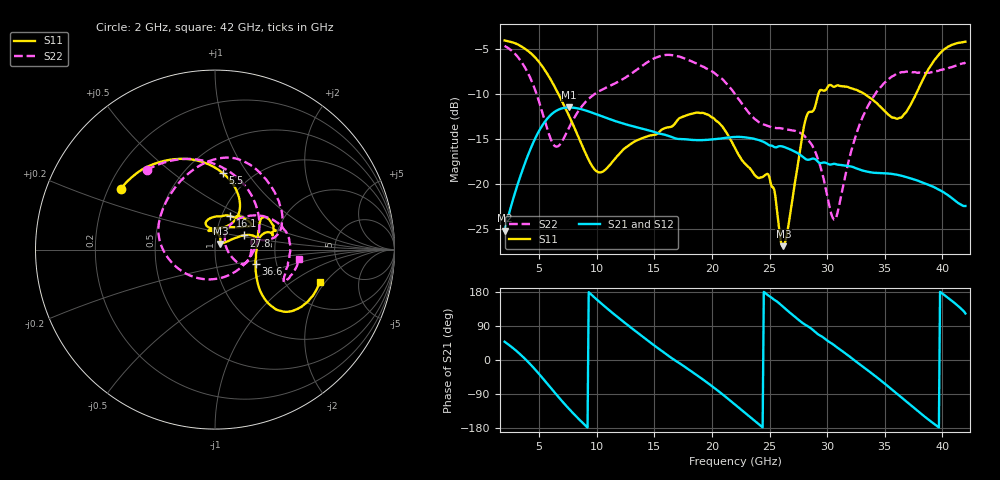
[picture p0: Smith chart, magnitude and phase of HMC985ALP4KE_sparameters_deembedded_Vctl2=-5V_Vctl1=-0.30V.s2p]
!s2p File: Measurements: S11, S21, S12, S22
# GHz S dB R 50.0
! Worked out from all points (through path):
!   401 points, 2 GHz to 42 GHz, reference 50 ohm
!   highest |S21| = -11.51 dB at 7.6 GHz (marker M1); lowest = -25.2 dB at 2 GHz (marker M2)
!   lowest |S11| = -26.9 dB at 26.2 GHz (marker M3), VSWR 1.09, Z = 52.9 + j3.6 ohm
!   |S11| at or under -10 dB: 6.664 GHz to 29.24 GHz (22.58 GHz wide, 126 % of centre); 33.21 GHz to 37.73 GHz (4.512 GHz wide, 12.7 % of centre)
!   |S22| runs from -24.0 to -4.7 dB; largest |S21 - S12| = 0.00026
!   S11 on the Smith chart (normalised r, x): 2 GHz: 0.25, +0.28; 5.5 GHz: 0.75, +0.78; 16.1 GHz: 1.10, +0.43; 27.8 GHz: 1.36, +0.22; 36.6 GHz: 1.56, -0.26; 42 GHz: 3.05, -1.80
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2  -4.08 147.2  -25.19 48.2  -25.19 48.2  -4.68 130.7
3.6  -4.86 120.5  -18.29 8.1  -18.29 8.1  -6.73 85.3
5.5  -7.38 84.0  -13.09 -55.1  -13.10 -55.1  -13.04 2.1
6.5  -9.59 67.0  -11.87 -91.4  -11.87 -91.4  -15.87 -71.2
7.6  -12.47 56.5  -11.51 -129.3  -11.51 -129.3  -13.74 -137.6
8.7  -15.66 58.8  -11.72 -163.6  -11.73 -163.6  -11.39 -171.4
10.2  -18.72 87.3  -12.37 154.2  -12.38 154.2  -9.71 164.3
11.9  -16.75 110.0  -13.15 111.1  -13.15 111.1  -8.64 141.1
15.4  -14.27 76.5  -14.41 29.3  -14.42 29.3  -5.86 87.2
16.1  -13.74 65.2  -14.61 13.8  -14.62 13.8  -5.68 78.5
19.4  -12.21 34.5  -15.12 -55.5  -15.13 -55.5  -7.10 35.6
22  -16.00 52.1  -14.79 -117.5  -14.79 -117.5  -10.03 10.5
24.9  -18.95 102.8  -15.65 170.1  -15.66 170.1  -13.60 13.0
26.2  -26.91 48.7  -15.87 139.6  -15.88 139.6  -13.88 -1.7
27.8  -15.01 26.4  -16.91 99.2  -16.91 99.2  -14.45 -22.7
28.7  -11.98 12.4  -17.20 81.0  -17.20 81.0  -15.72 -29.0
30.7  -9.19 20.4  -17.78 36.8  -17.79 36.8  -23.93 23.3
32.9  -9.78 33.7  -18.44 -13.2  -18.45 -13.1  -13.14 51.9
35.4  -12.39 11.1  -18.86 -72.3  -18.86 -72.3  -8.31 21.7
36.6  -12.40 -19.5  -19.14 -102.7  -19.15 -102.7  -7.59 6.7
39.5  -5.96 -42.8  -20.50 -173.4  -20.50 -173.4  -7.47 -24.6
42  -4.22 -17.3  -22.45 122.7  -22.46 122.7  -6.51 -6.2
